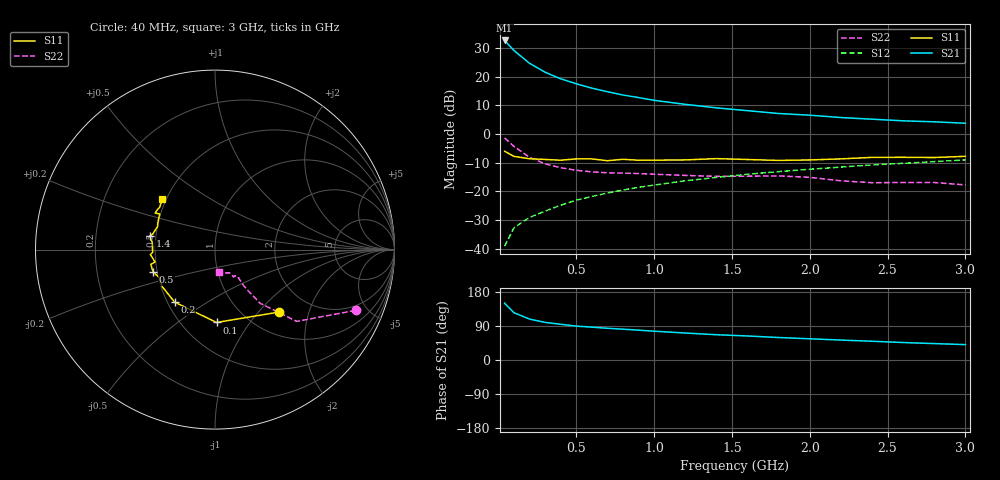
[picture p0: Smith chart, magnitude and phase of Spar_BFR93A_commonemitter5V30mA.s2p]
! Filename:  BFR93AD.S2P  Version:  2.0
! NXP part #: BFR93A  Date: May 1990
! Bias condition: Vce=5V, Ic=30mA
#  MHz  S  MA  R  50
! Freq  S11  S21  S12  S22  !GUM [dB]
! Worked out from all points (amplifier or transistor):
!   21 points, 40 MHz to 3 GHz, reference 50 ohm
!   highest |S21| = 32.6 dB at 40 MHz (marker M1)
!   |S21| within 3 dB of that: start of sweep to 91.47 MHz
!   unconditionally stable (mu >= 1): 645.8 MHz to 2.847 GHz
!   at 300 MHz: K = 0.90, MSG = 24.2 dB, |S12| = -26.9 dB
!   at 1 GHz: K = 1.04, MAG = 13.6 dB, |S12| = -17.9 dB
!   at 3 GHz: K = 0.99, MSG = 6.4 dB, |S12| = -9.1 dB
!   S11 on the Smith chart (normalised r, x): 40 MHz: 1.41, -1.30; 100 MHz: 0.73, -0.71; 200 MHz: 0.54, -0.37; 500 MHz: 0.47, -0.14; 1.4 GHz: 0.46, +0.08; 3 GHz: 0.48, +0.32
40  0.499 -44.2  42.81 149.9  0.011 74.3  0.853 -23.4
100  0.406 -88.8  28.62 124.9  0.023 62.9  0.606 -41.3
200  0.369 -127.6  17.1 107.9  0.035 64.2  0.392 -49.9
300  0.359 -144.5  11.93 99.3  0.045 66.9  0.301 -51.1
400  0.348 -153.5  9.173 94.3  0.057 68.3  0.257 -51.5
500  0.367 -160.2  7.512 89.4  0.07 70.5  0.232 -50.9
600  0.367 -167.0  6.297 86.7  0.081 70.8  0.218 -50.7
700  0.341 -168.3  5.464 83.7  0.093 72.8  0.21 -50.7
800  0.361 -175.7  4.781 81.3  0.105 72.0  0.207 -49.9
900  0.348 -177.4  4.317 78.8  0.117 72.3  0.204 -50.4
1000  0.349 176.8  3.861 76.0  0.128 72.3  0.198 -49.9
1200  0.352 173.4  3.286 71.2  0.152 71.5  0.189 -50.8
1400  0.371 168.3  2.852 66.7  0.174 70.2  0.182 -53.4
1600  0.358 166.1  2.548 63.4  0.198 69.2  0.183 -54.4
1800  0.345 158.4  2.273 59.3  0.22 68.0  0.185 -56.0
2000  0.352 154.7  2.126 56.0  0.242 66.5  0.175 -56.0
2200  0.367 147.1  1.932 52.6  0.264 66.2  0.152 -58.2
2400  0.39 148.6  1.81 49.5  0.288 64.1  0.141 -67.2
2600  0.391 146.3  1.694 46.1  0.307 62.5  0.142 -74.4
2800  0.388 142.6  1.628 43.3  0.329 61.4  0.142 -78.4
3000  0.407 136.2  1.537 40.6  0.352 59.2  0.129 -80.1
